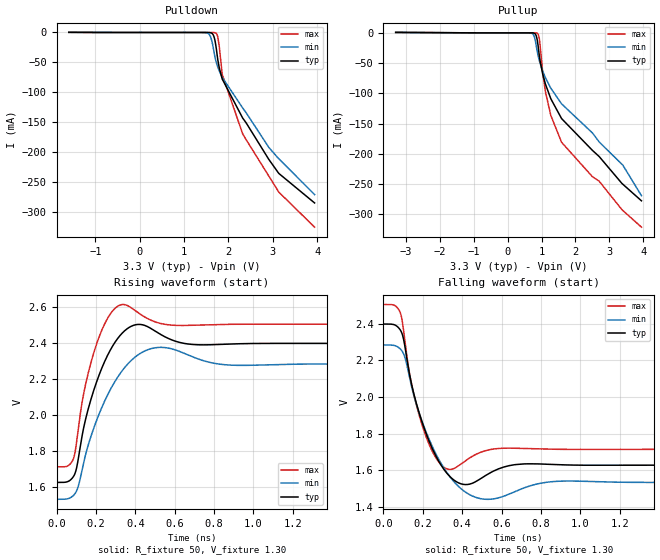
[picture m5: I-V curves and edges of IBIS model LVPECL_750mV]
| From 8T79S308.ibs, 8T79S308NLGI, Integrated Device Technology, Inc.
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[Model]   LVPECL_750mV
Model_type   Output_ECL
Polarity   Non-Inverting
|   typ   min   max
C_comp   2pF   1.5pF   2.5pF
Vmeas= 2.000V
Rref = 50
Cref = 0
Vref = 1.3V
|   typ   min   max
[Voltage range]   3.3V   3.135V   3.465V
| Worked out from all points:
|   rising waveform, R_fixture 50, V_fixture 1.30: 20-80 % time 110ps typ, 142ps min, 84.9ps max; typ from 1.63 V to 2.4 V
|   falling waveform, R_fixture 50, V_fixture 1.30: 20-80 % time 110ps typ, 142ps min, 84.9ps max; typ from 2.4 V to 1.63 V
[Pulldown]
|Voltage   I (typ)   I (min)   I (max)
|Note, modeling breaks down at 250mA and above.  This is well beyond the functional   |
|operating range of the device.  Should this scenario occur, catastrophic failure and   |
|possible damage to the device and/or board is of higher concern than the I-V curve   |
|behavior.  The IBIS checker will flag currents in excess of 10A with warnings.  Lines   |
|with currents in excess of 0.35 A have been commented out.  The points still remain|
|available to the user if the user desires to use them.   |
-1.6V     225.4uA    213.6uA    245.6uA
1.5V      -11.49uA   -434.3uA   -27.56nA
1.598V    -473.3uA   -7.549mA   -3.342uA
1.664V    -5.004mA   -28.01mA   -81.52uA
1.713V    -20.18mA   -46.31mA   -879.4uA
1.762V    -46.5mA    -58.31mA   -7.992mA
1.795V    -59.7mA    -64.63mA   -24.46mA
1.86V     -77.96mA   -75.14mA   -70.43mA
2.32V     -143mA     -126.2mA   -169.3mA
2.91V     -212.3mA   -192.2mA   -240.1mA
3.14V     -236.1mA   -211.5mA   -267.4mA
3.943V    -285.3mA   -271.3mA   -325.8mA
| 4.14000e+00   -3.02896e-01   -3.87853e-01   -3.44619e-01
| 4.22200e+00   -3.46819e-01   -4.37187e-01   -3.53806e-01
| 4.41880e+00   -4.88381e-01   -5.56882e-01   -3.86188e-01
| 4.53360e+00   -5.72163e-01   -6.27224e-01   -4.90345e-01
| 4.55000e+00   -5.84213e-01   -6.37295e-01   -5.05646e-01
| 4.71400e+00   -7.05444e-01   -7.38306e-01   -6.58457e-01
| 5.22240e+00   -1.08526e+00   -9.93910e-01   -1.13890e+00
| 5.51760e+00   -1.33394e+00   -9.93910e-01   -1.42071e+00
| 5.94400e+00   -1.34850e+00   -9.93910e-01   -1.85853e+00
| 5.96040e+00   -1.34850e+00   -9.93910e-01   -1.87645e+00
[Pullup]
|Voltage   I (typ)   I (min)   I (max)
|Note, modeling breaks down at 250mA and above.  This is well beyond the functional   |
|operating range of the device.  Should this scenario occur, catastrophic failure and   |
|possible damage to the device and/or board is of higher concern than the I-V curve   |
|behavior.  The IBIS checker will flag currents in excess of 10A with warnings.  Lines   |
|with currents in excess of 0.35 A have been commented out.  The points still remain|
|available to the user if the user desires to use them.   |
-3.3V     763.6uA    674.5uA    902.1uA
679.8mV   -11.35uA   -275.3uA   -54.15nA
778.8mV   -476.8uA   -5.126mA   -6.729uA
877.8mV   -13.01mA   -32.07mA   -815.5uA
937.2mV   -38.81mA   -46.33mA   -10.53mA
1.036V    -68.41mA   -63.43mA   -66.62mA
1.115V    -84.76mA   -74.19mA   -97.29mA
1.274V    -109mA     -91.55mA   -136.6mA
1.591V    -141.7mA   -117.4mA   -181mA
2.699V    -204.6mA   -180.4mA   -245.4mA
3.392V    -250.2mA   -218.4mA   -293.7mA
3.947V    -277.9mA   -269.4mA   -321.4mA
| 4.10520e+00   -2.91375e-01   -3.64699e-01   -3.35506e-01
| 4.22400e+00   -3.42994e-01   -4.36855e-01   -3.47946e-01
| 4.38240e+00   -4.58790e-01   -5.33732e-01   -3.67801e-01
| 4.67940e+00   -6.78568e-01   -7.16900e-01   -6.20872e-01
| 4.69920e+00   -6.93305e-01   -7.29163e-01   -6.39605e-01
| 4.85760e+00   -8.11485e-01   -8.28324e-01   -7.89901e-01
| 4.91700e+00   -8.55918e-01   -8.67590e-01   -8.46402e-01
| 5.07540e+00   -9.74550e-01   -9.82239e-01   -9.97314e-01
| 5.15460e+00   -1.03400e+00   -9.82239e-01   -1.07287e+00
| 5.53080e+00   -1.34585e+00   -9.82239e-01   -1.43239e+00
| 5.94660e+00   -1.34585e+00   -9.82239e-01   -1.86160e+00
| 5.96640e+00   -1.34585e+00   -9.82239e-01   -1.88324e+00
[Ramp]
|   typ   min   max
dV/dt_r   0.525/0.14n   0.505/0.177n   0.539/0.109n
dV/dt_f   0.525/0.14n   0.505/0.177n   0.539/0.109n
R_load =   50.0000
[Rising Waveform]
R_fixture = 50
V_fixture = 1.30   | VCC_typ - 2V
V_fixture_max = 1.465   | VCC_max - 2V
V_fixture_min = 1.135   | VCC_min - 2V
C_fixture = 0.0p
| Time   typ   min   max
0s        1.628V     1.534V     1.714V
86.09ps   1.661V     1.556V     1.76V
136.1ps   1.922V     1.729V     2.11V
188.2ps   2.135V     1.926V     2.343V
254.3ps   2.321V     2.101V     2.527V
322.3ps   2.442V     2.23V      2.611V
414.4ps   2.504V     2.335V     2.569V
524.5ps   2.451V     2.376V     2.51V
878.9ps   2.395V     2.278V     2.504V
2ns       2.398V     2.284V     2.504V
[Falling Waveform]
R_fixture = 50
V_fixture = 1.30   | VCC_typ - 2V
V_fixture_max = 1.465   | VCC_max - 2V
V_fixture_min = 1.135   | VCC_min - 2V
C_fixture = 0.0p
| Time   typ   min   max
0s        2.398V     2.284V     2.504V
86.09ps   2.365V     2.262V     2.459V
136.1ps   2.104V     2.089V     2.109V
188.2ps   1.891V     1.892V     1.876V
254.3ps   1.705V     1.717V     1.691V
322.3ps   1.584V     1.588V     1.608V
416.4ps   1.522V     1.481V     1.652V
524.5ps   1.575V     1.442V     1.709V
878.9ps   1.631V     1.54V      1.715V
2ns       1.628V     1.534V     1.714V
